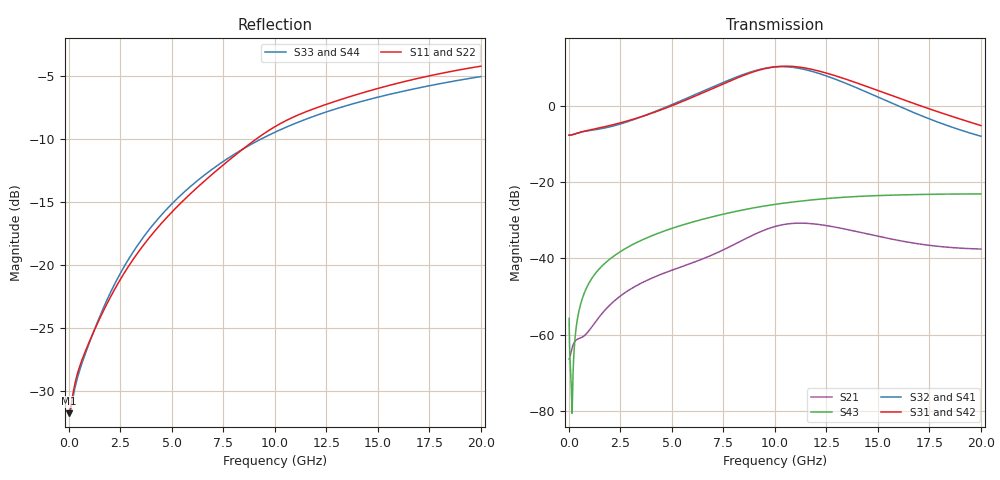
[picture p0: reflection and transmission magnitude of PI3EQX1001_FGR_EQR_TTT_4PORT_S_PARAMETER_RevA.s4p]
! NPort=4 DATA=2000 NOISE=0 GROUPDELAY=0 COMPLEX_DATAFORMAT=POLAR
! NumOfBlock=1 NumOfParam=0
! .MODEL Smodel S TSTONEFILE=PI3EQX1001_FGR_EQR_TTT_4PORT_S_PARAMETER_RevA.s4p TYPE=S
!  -- The above .MODEL line can be used for the S element in the netlist.
! The s parameter is extracted from the linear redriver, it is not bi-directional; only s(4,1)s(4,2) and s(3,1)s(3,2)
! should be the insertion loss
!Port definition:
!Port1 = input+
!Port2 = input¨C
!Port3 = output+
!Port4 = output-
# Hz S MA R  50
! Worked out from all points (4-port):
!   2000 points, 10 MHz to 20 GHz, reference 50 ohm
!   strongest paths, dB at 10 MHz, 5.01 GHz, 10.01 GHz, 15.01 GHz, 20 GHz:
!     S31: -7.6, 0.2, 10.4, 4.1, -5.1
!     S42: -7.6, 0.1, 10.4, 4.1, -5.1
!     S32: -7.6, 0.5, 10.3, 2.4, -7.9
!     S41: -7.6, 0.4, 10.3, 2.3, -7.9
!     S43: -55.8, -32.1, -25.8, -23.5, -23.1
!     S21: -66.4, -43.1, -31.6, -34.2, -37.5
!   lowest |S11| = -31.7 dB at 10 MHz (marker M1), VSWR 1.05, Z = 47.5 - j0.063 ohm
!   |S11| at or under -10 dB: start of sweep to 9.111 GHz
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1e7  0.0259 -178.5  0.0004911 2.7  3.669e-05 -0.2  4.787e-05 -0.1
     0.0004778 2.9  0.02597 -178.7  4.577e-05 -0.2  5.994e-05 -0.1
     0.4169 -0.3  0.4169 179.7  0.02616 178.4  0.001615 -59.2
     0.4167 179.7  0.4168 -0.3  0.001626 -59.0  0.02612 178.4
7.47e9  0.2483 -106.1  0.01218 77.6  2.144e-05 -30.9  3.196e-05 -29.8
        0.01286 75.7  0.2463 -106.0  2.87e-05 -25.1  3.947e-05 -25.1
        1.958 -59.4  2.044 126.6  0.2566 -112.3  0.03808 54.1
        2.035 126.7  1.955 -59.4  0.03804 54.2  0.2563 -112.3
9.48e9  0.3319 -108.6  0.02259 58.8  1.935e-05 -27.4  3.391e-05 -34.2
        0.02352 57.2  0.3295 -108.6  3.138e-05 -26.5  3.732e-05 -23.8
        3.108 -115.1  3.138 70.6  0.32 -115.2  0.04883 41.3
        3.123 70.8  3.103 -115.1  0.04882 41.3  0.3199 -115.2
1.114e10  0.3932 -113.2  0.028 27.2  2.217e-05 -19.9  3.523e-05 -47.8
          0.02908 26.0  0.3902 -113.3  3.314e-05 -39.3  4.035e-05 -21.2
          3.281 -172.8  3.161 13.5  0.368 -118.0  0.05628 30.1
          3.144 13.7  3.275 -172.9  0.05623 30.0  0.3677 -118.0
1.349e10  0.4602 -118.5  0.02306 -6.1  3.05e-05 -37.7  2.969e-05 -72.1
          0.02406 -7.1  0.4564 -118.5  2.755e-05 -61.4  4.813e-05 -34.2
          2.247 117.6  1.978 -53.5  0.428 -122.0  0.06417 14.3
          1.967 -53.1  2.242 117.6  0.06405 14.3  0.428 -122.0
1.598e10  0.5251 -123.1  0.01642 -18.9  3.002e-05 -71.7  2.084e-05 -103.2
          0.01729 -20.2  0.5208 -123.1  1.796e-05 -88.0  4.471e-05 -58.0
          1.29 63.3  1.01 -101.4  0.4827 -125.8  0.06835 -1.3
          1.005 -100.8  1.287 63.3  0.06825 -1.2  0.4824 -125.7
2e10  0.6129 -130.1  0.01269 -16.0  1.728e-05 -144.4  1.48e-05 145.1
      0.01328 -18.6  0.6075 -130.2  9.969e-06 129.4  2.054e-05 -96.8
      0.5575 -1.1  0.4034 -145.3  0.5574 -131.2  0.07044 -23.6
      0.4037 -144.4  0.5562 -1.1  0.07039 -23.6  0.5573 -131.1
